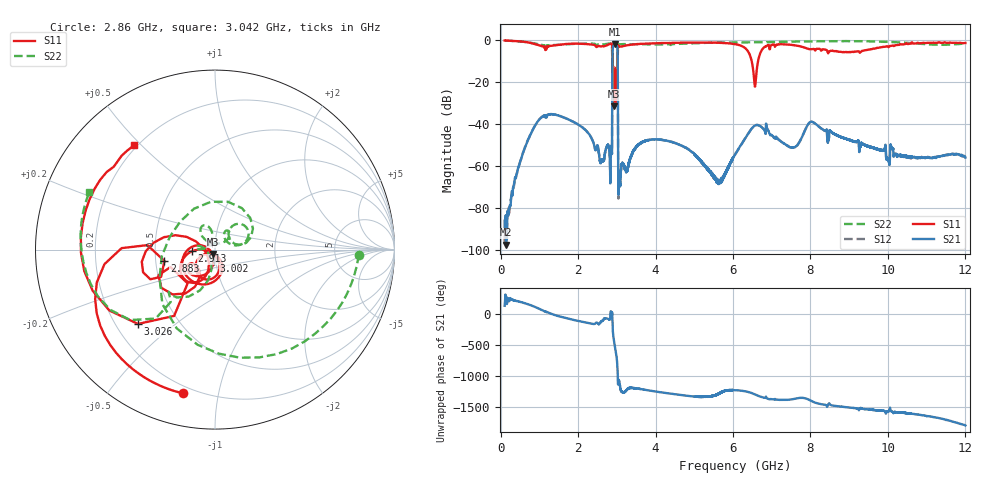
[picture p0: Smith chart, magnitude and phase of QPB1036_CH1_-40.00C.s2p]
! TDS: K:\Engsetup\Winsaw\QPB1036_ALL
! Channel 1
! Ports=1 2
! seg 1=100.000000 1100.000000 101
! seg 2=1101.000000 1501.000000 401
! seg 3=1502.000000 2502.000000 101
! seg 4=2503.000000 3803.000000 1301
! seg 5=3804.000000 5004.000000 121
! seg 6=5005.000000 6005.000000 1001
! seg 7=6006.000000 8406.000000 241
! seg 8=8407.000000 10607.000000 2201
! seg 9=10608.000000 12008.000000 141
! Points=5609
! FailCode=0
! Topology=ALL_SE(12)
!VNA Cal loaded =QPB1036_ALL_-40C
!PS1(V)= 5.000
!PS(mA)= 0.300
!PS2(V)= 0.630
!PS(mA)= -0.100
!PS3(V)= 0.630
!PS(mA)= 0.100
!PS4(V)= 1.170
!PS(mA)= -0.100
!Temp (C)= -40.00
# MHz S DB R 50
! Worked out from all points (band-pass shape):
!   5609 points, 100 MHz to 12.01 GHz, reference 50 ohm
!   highest |S21| = -2.14 dB at 2.95 GHz (marker M1); lowest = -97.5 dB at 140 MHz (marker M2)
!   |S21| within 3 dB of the highest: 2.891 GHz to 3.02 GHz (128.6 MHz wide, 4.35 % of centre)
!   lowest |S11| = -31.5 dB at 2.92 GHz (marker M3), VSWR 1.05, Z = 49 - j2.44 ohm
!   |S11| at or under -10 dB: 2.89 GHz to 3.019 GHz (129.9 MHz wide, 4.4 % of centre); 3.022341 GHz to 3.024458 GHz (2.117 MHz wide, 0.07 % of centre); 6.484 GHz to 6.651 GHz (166.8 MHz wide, 2.54 % of centre)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
!   |S22| runs from -29.4 to -0.3 dB; largest |S21 - S12| = 0.0079
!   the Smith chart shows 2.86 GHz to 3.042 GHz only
!   S11 on the Smith chart (normalised r, x): 2.86 GHz: 0.16, -0.79; 2.883 GHz: 0.56, -0.08; 2.913 GHz: 0.77, -0.02; 3.002 GHz: 0.98, -0.13; 3.026 GHz: 0.29, -0.37; 3.042 GHz: 0.19, +0.47
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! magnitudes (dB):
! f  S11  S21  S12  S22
! 100 MHz  -0.2  -86.2  -97.0  -0.3
! 140 MHz  -0.3  -97.5  -98.3  -0.3
! 1.121 GHz  -3.7  -36.2  -36.3  -3.1
! 2.092 GHz  -1.8  -41.4  -41.4  -1.8
! 2.582 GHz  -3.1  -58.8  -58.3  -2.2
! 2.846 GHz  -1.8  -54.5  -54.3  -1.7
! 2.86 GHz  -1.7  -50.3  -50.4  -1.9
! 2.883 GHz  -10.8  -13.4  -13.4  -11.7
! 2.913 GHz  -17.7  -2.6  -2.6  -16.8
! 2.92 GHz  -31.5  -2.4  -2.4  -21.9
! 2.95 GHz  -20.0  -2.1  -2.1  -23.5
! 3.002 GHz  -23.8  -2.8  -2.8  -27.1
! 3.026 GHz  -4.5  -16.8  -16.8  -4.2
! 3.042 GHz  -2.7  -73.8  -73.3  -2.3
! 3.068 GHz  -3.2  -66.4  -65.6  -2.1
! 3.513 GHz  -2.0  -50.7  -50.9  -2.0
! 4.074 GHz  -1.5  -47.4  -47.5  -2.1
! 5.633 GHz  -1.3  -67.3  -67.2  -1.2
! 6.056 GHz  -2.0  -54.6  -54.7  -1.2
! 8.046 GHz  -4.4  -39.0  -39.0  -0.6
! 10.02 GHz  -3.4  -57.4  -57.4  -0.9
! 12.01 GHz  -1.5  -56.1  -56.1  -1.7
